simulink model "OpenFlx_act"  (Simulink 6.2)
settings: Solver=ode45  StartTime=0.0  StopTime=10.0  RelTol=1e-3
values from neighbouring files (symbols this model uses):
  Kp = om^2*Iy/(l*T)    (= 0.554556771732)    [run.m]    (also in run3.m = 0.554540604935)
  Kr = 2*0.85*om*Iy/(l*T)    (= 1.03530256089)    [run.m]    (also in run3.m = 1.03527237908)
  wd = 7    [run.m]    (also in run3.m)
  wd2 = 16    [run.m]    (also in run3.m)
  wf = 9    [run.m]    (also in run3.m)
  wn = 7.4    [run.m]    (also in run3.m)
  wn2 = 16.8    [run.m]    (also in run3.m)
  zd = 0.2    [run.m]    (also in run3.m)
  zd2 = 0.2    [run.m]    (also in run3.m)
  zn = 0.02    [run.m]    (also in run3.m)
  zn2 = 0.015    [run.m]    (also in run3.m)
undefined symbols (not defined in the file or in its folder): Ava, Bva, Cva, Dva

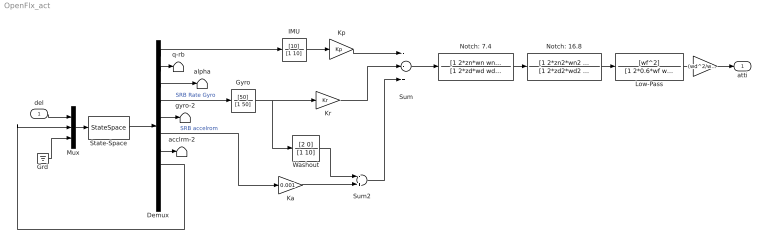
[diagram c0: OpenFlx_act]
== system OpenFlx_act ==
  del : Inport  Port=1  LatchInput=off
  " " : Gain  Gain=(wd^2/wn^2)*(wd2^2/wn2^2)
  Demux : Demux  Outputs=10
  Grd : Ground
  Gyro : TransferFcn  Numerator=[50]  Denominator=[1 50]
  IMU : TransferFcn  Numerator=[10]  Denominator=[1 10]
  Ka : Gain  Gain=0.001
  Kp : Gain  Gain=Kp
  Kr : Gain  Gain=Kr
  Low-Pass : TransferFcn  Numerator=[wf^2]  Denominator=[1 2*0.6*wf wf^2]
  Mux : Mux  Inputs=3
  Notch: 16.8 : TransferFcn  Numerator=[1 2*zn2*wn2 wn2^2]  Denominator=[1 2*zd2*wd2 wd2^2]
  Notch: 7.4 : TransferFcn  Numerator=[1 2*zn*wn wn^2]  Denominator=[1 2*zd*wd wd^2]
  State-Space : StateSpace  A=Ava  B=Bva  C=Cva  D=Dva
  Sum : Sum  Inputs=--+
  Sum2 : Sum  Inputs=-+
  Washout : TransferFcn  Numerator=[2 0]  Denominator=[1 10]
  acclrm-2 : Terminator
  alpha : Terminator
  gyro-2 : Terminator
  q-rb : Terminator
  atti : Outport
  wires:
  Mux/1 -> State-Space/1
  del/1 -> Mux/1
  Demux/4 -> Gyro/1  "SRB Rate Gyro"
  Demux/6 -> Ka/1  "SRB accelrom"
  Kp/1 -> Sum/1
  Kr/1 -> Sum/2
  Demux/7 -> acclrm-2/1
  Ka/1 -> Sum2/2
  Sum2/1 -> Sum/3
  State-Space/1 -> Demux/1
  Demux/1 -> IMU/1
  Demux/2 -> q-rb/1
  Demux/3 -> alpha/1
  Demux/5 -> gyro-2/1
  IMU/1 -> Kp/1
  Gyro/1 -> Washout/1, Kr/1
  Demux/8 -> Mux/2
  Grd/1 -> Mux/3
  Notch: 7.4/1 -> Notch: 16.8/1
  Notch: 16.8/1 -> Low-Pass/1
  " "/1 -> atti/1
  Sum/1 -> Notch: 7.4/1
  Low-Pass/1 -> " "/1
  Washout/1 -> Sum2/1
